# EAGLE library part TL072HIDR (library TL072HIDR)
Dual-channel low input bias current standard op amp Source: Datasheet
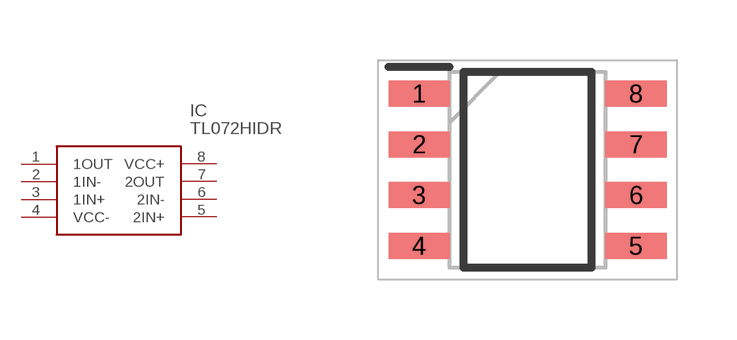
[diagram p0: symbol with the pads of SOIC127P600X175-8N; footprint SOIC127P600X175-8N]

Designator prefix IC

## TL072HIDR (Arrow_Part_Number: TL072HIDR; Arrow_Price-Stock: https://www.arrow.com/en/products/tl072hidr/texas-instruments?utm_currency=USD&region=nac; Description: Dual-channel low input bias current standard op amp; Height: 1.75mm; Manufacturer_Name: Texas Instruments; Manufacturer_Part_Number: TL072HIDR; Mouser_Part_Number: 595-TL072HIDR; Mouser_Price-Stock: https://www.mouser.co.uk/ProductDetail/Texas-Instruments/TL072HIDR?qs=aP1CjGhiNiHyZHNBkxIRdA%3D%3D)  [SOIC127P600X175-8N]
1  1OUT
2  1IN-
3  1IN+
4  VCC-
5  2IN+
6  2IN-
7  2OUT
8  VCC+

## Footprint SOIC127P600X175-8N (pad centres in mm)
D(R-PDSO-G)
smd 1.528 x 0.65: 1 -2.711,1.905; 2 -2.711,0.635; 3 -2.711,-0.635; 4 -2.711,-1.905; 5 2.711,-1.905; 6 2.711,-0.635; 7 2.711,0.635; 8 2.711,1.905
